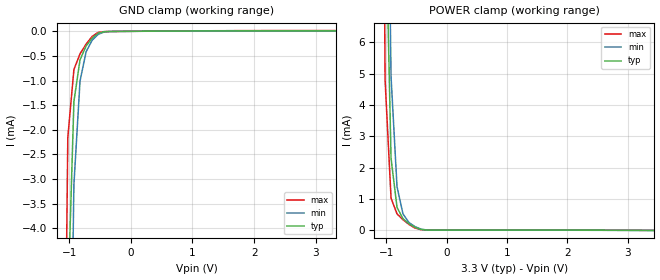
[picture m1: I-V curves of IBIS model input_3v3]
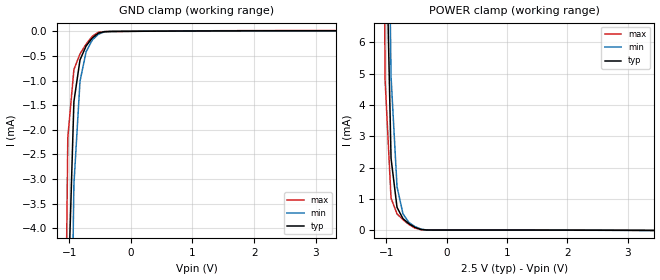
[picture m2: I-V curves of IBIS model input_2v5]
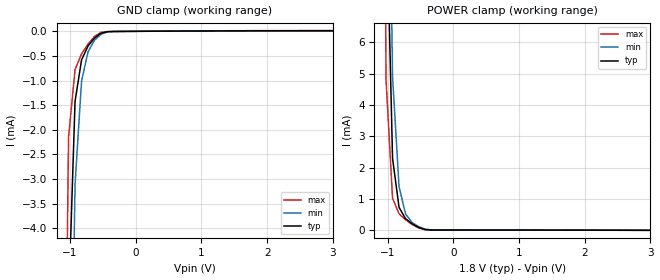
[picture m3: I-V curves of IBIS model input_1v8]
[IBIS ver]   4.1
[File name]   551s.ibs
|[File Rev]   1.0
|[Date]   March  3rd, 2016
[File Rev]   1.0
[Date]   April 25th, 2016[Source]   IDT
[Notes]   1. Temp typ=55C, min=80C, max=-40C
[Disclaimer]
READ THESE TERMS AND CONDITIONS CAREFULLY BEFORE USING THIS IBIS MODEL.  BY
USING THIS IBIS MODEL, YOU ARE ACCEPTING AND AGREEING TO THESE TERMS AND
CONDITIONS OF USE.
INTEGRATED DEVICE TECHNOLOGY, INC. ("IDT") HEREBY GRANTS THE USER OF THIS
IBIS MODEL ("USER") A NON-EXCLUSIVE, NONTRANSFERABLE LICENSE TO USE THIS
IBIS MODEL UNDER THE FOLLOWING TERMS: THE USER IS GRANTED THIS LICENSE ONLY
TO USE THE IBIS MODEL FOR DEMONSTRATION PURPOSES ONLY AND IS NOT GRANTED
RIGHTS TO SELL, COPY (EXCEPT AS NEEDED TO RUN THE IBIS MODEL), RENT, LEASE
OR SUB-LICENSE (EXCEPT FOR DEMONSTRATION) THE IBIS MODEL IN WHOLE OR IN
PART, OR IN MODIFIED FORM TO ANYONE. THE USER MAY MODIFY THE IBIS MODEL TO
SUIT ITS SPECIFIC APPLICATIONS, BUT  RIGHTS TO DERIVATIVE WORKS AND SUCH
MODIFICATIONS SHALL BELONG TO IDT.
THIS IBIS MODEL IS PROVIDED ON AN AS IS" BASIS AND IDT  MAKES ABSOLUTELY NO
WARRANTY WITH RESPECT TO THE INFORMATION CONTAINED HEREIN.  IDT DISCLAIMS
AND USER WAIVES ALL WARRANTIES, EXPRESS AND IMPLIED, INCLUDING WARRANTIES OF
MERCHANTABILITY AND FITNESS FOR A PARTICULAR PURPOSE.  THE ENTIRE RISK AS TO
QUALITY AND PERFORMANCE IS WITH THE USER  ACCORDINGLY, IN NO EVENT SHALL IDT
BE LIABLE FOR ANY DIRECT OR INDIRECT DAMAGES, WHETHER IN CONTRACT OR TORT,
INCLUDING ANY LOST PROFITS OR OTHER INCIDENTAL, CONSEQUENTIAL, EXEMPLARY, OR
PUNITIVE DAMAGES ARISING OUT OF THE USE OR APPLICATION OF THE  IBIS MODEL,
WHETHER OR NOT IDT HAD NOTICE OF SUCH DAMAGES.
IDT RESERVES THE RIGHT TO MAKE CHANGES WITHOUT NOTICE TO ANY PRODUCT HEREIN
TO IMPROVE RELIABILITY, FUNCTION, OR DESIGN. IDT DOES NOT CONVEY ANY LICENSE
UNDER PATENT RIGHTS OR ANY OTHER INTELLECTUAL PROPERTY RIGHTS, INCLUDING
THOSE OF THIRD PARTIES. IDT IS NOT OBLIGATED TO PROVIDE  MAINTENANCE OR
SUPPORT FOR THE LICENSED IBIS MODEL.
This model is for  IDT Fan Out Buffer
[Copyright]
Copyright 2002, Integrated Device Technology, Inc. All rights  reserved.
|History
|Rev 1.0 Created on April 25th, 2016
|   Component 551S
[Component]   551S
[Manufacturer]   Integrated Device Technology Inc.
[Package]
| Following package parameters are for the 8 pin DFN package (cmg_8)
| variable   typ   min   max
R_pkg   72.4655m   58.886m   86.045m
L_pkg   1.47175nH   1.11650nH   1.77850nH
C_pkg   0.07747pF   0.07444pF   0.08050pF
[Pin]  signal_name   model_name
1   ICLK   cmos_input
2   Q1   lvcmos
3   Q2   lvcmos
4   Q3   lvcmos
5   Q1   lvcmos
6   GND   gnd
7   VDD   POWER
8   OE   cmos_input
[Model Selector] lvcmos
lvcmos_3v3   3.3v cmos
lvcmos_2v5   2.5v cmos
lvcmos_1v8   1.8v cmos
[Model Selector] cmos_input
input_3v3  3.3v cmos
input_2v5  2.5v cmos
input_1v8  1.8v cmos
| Models and submodels in the file (6): input_3v3 (Input), input_2v5 (Input), input_1v8 (Input), lvcmos_3v3 (Output), lvcmos_2v5 (Output), lvcmos_1v8 (Output)
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|   Model INPUT_3V3
[Model]   input_3v3
Model_type   Input
Polarity   Non-Inverting
Vinl = 0.8V
Vinh = 2.0V
|   typ   min   max
C_comp   2pF   1.5pF   2.5pF
|   typ   min   max
[Voltage range]   3.3V   3.135V   3.465V
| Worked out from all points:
|   GND clamp passes 1 mA (typ) near -0.87 V on its own axis
|   POWER clamp passes 1 mA (typ) near -0.84 V on its own axis
[GND_clamp]
|Voltage   I (typ)   I (min)   I (max)
-3.3V     -5.877A    -5.408A    -6.492A
-1.122V   -26.71mA   -42.1mA    -13.37mA
-1.023V   -5.55mA    -11.5mA    -2.155mA
-924mV    -1.425mA   -3.112mA   -776.1uA
-825mV    -579.5uA   -1.011mA   -457.9uA
-726mV    -298.2uA   -414.7uA   -259.6uA
-627mV    -135.7uA   -178.7uA   -102.9uA
-528mV    -37.47uA   -59.22uA   -19.83uA
-429mV    -6.866uA   -11.92uA   -5.643uA
-330mV    -3.062uA   -3.056uA   -3.933uA
3.333V    11.06uA    8.259uA    15.61uA
| 3.43200e+00   1.10646e-05   9.85198e-06   1.56123e-05
| 3.46500e+00   1.10748e-05   1.56686e-05   1.56145e-05
| 3.53100e+00   1.10953e-05   2.73017e-05   1.56184e-05
| 3.63000e+00   1.22240e-05   9.00221e-05   1.56239e-05
| 3.72900e+00   2.94089e-05   2.01383e-04   1.56343e-05
| 3.82800e+00   9.82853e-05   4.04552e-04   1.61859e-05
| 3.92700e+00   2.13921e-04   9.74740e-04   3.14030e-05
| 4.02600e+00   3.75114e-04   3.15078e-03   1.08238e-04
| 4.12500e+00   7.35643e-04   1.23144e-02   2.36650e-04
| 4.22400e+00   2.30231e-03   4.64533e-02   3.97348e-04
| 4.32300e+00   1.10342e-02   1.34572e-01   6.21132e-04
| 4.42200e+00   5.26801e-02   2.82717e-01   1.53968e-03
| 4.52100e+00   1.68112e-01   4.72773e-01   9.44647e-03
| 4.62000e+00   3.53430e-01   6.87934e-01   6.47105e-02
| 4.71900e+00   5.79768e-01   9.19142e-01   2.25514e-01
| 4.81800e+00   8.28544e-01   1.16053e+00   4.62411e-01
| 4.91700e+00   1.09117e+00   1.40901e+00   7.35436e-01
| 5.01600e+00   1.36245e+00   1.66266e+00   1.02689e+00
| 5.11500e+00   1.63974e+00   1.92021e+00   1.32900e+00
| 5.21400e+00   1.92140e+00   2.18081e+00   1.63813e+00
| 5.31300e+00   2.20638e+00   2.44384e+00   1.95201e+00
| 5.41200e+00   2.49395e+00   2.70886e+00   2.26936e+00
| 5.51100e+00   2.78359e+00   2.97552e+00   2.58936e+00
| 5.61000e+00   3.07492e+00   3.24357e+00   2.91142e+00
| 5.70900e+00   3.36767e+00   3.51280e+00   3.23516e+00
| 5.80800e+00   3.66160e+00   3.78306e+00   3.56026e+00
| 5.90700e+00   3.95656e+00   4.05420e+00   3.88650e+00
| 6.00600e+00   4.25239e+00   4.32613e+00   4.21370e+00
| 6.10500e+00   4.54899e+00   4.59875e+00   4.54174e+00
| 6.20400e+00   4.84627e+00   4.87198e+00   4.87049e+00
| 6.30300e+00   5.14414e+00   5.14577e+00   5.19987e+00
| 6.40200e+00   5.44256e+00   5.42005e+00   5.52980e+00
| 6.50100e+00   5.74145e+00   5.69479e+00   5.86022e+00
| 6.60000e+00   6.04077e+00   5.96994e+00   6.19109e+00
[Power_clamp]
|Voltage   I (typ)   I (min)   I (max)
-3.3V     6.041A     5.512A     6.743A
-1.122V   52.68mA    68.73mA    36.05mA
-1.023V   11.03mA    19.49mA    4.811mA
-924mV    2.302mA    4.908mA    1.028mA
-825mV    735.6uA    1.396mA    528.4uA
-726mV    375.1uA    526.2uA    340.6uA
-627mV    213.9uA    252.9uA    189.6uA
-528mV    98.2uA     121.6uA    75.41uA
-429mV    29.41uA    42.52uA    21.55uA
-231mV    11.1uA     8.404uA    15.63uA
3.432V    -1.145uA   -2.375uA   378.6nA
|   Model INPUT_2V5
[Model]   input_2v5
Model_type Input
Vinl =   0.9500V
Vinh =   1.5500V
C_comp   2.0000pF   1.5000pF   2.5000pF
[Temperature Range]   55.0000   80.0000   -40.0000
[Voltage Range]   2.5000V   2.3750V   2.6250V
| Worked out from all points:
|   GND clamp passes 1 mA (typ) near -0.87 V on its own axis
|   POWER clamp passes 1 mA (typ) near -0.84 V on its own axis
[GND_clamp]
|Voltage   I (typ)   I (min)   I (max)
-3.3V     -5.877A    -5.408A    -6.492A
-1.122V   -26.71mA   -42.1mA    -13.37mA
-1.023V   -5.55mA    -11.5mA    -2.155mA
-924mV    -1.425mA   -3.112mA   -776.1uA
-825mV    -579.5uA   -1.011mA   -457.9uA
-726mV    -298.2uA   -414.7uA   -259.6uA
-627mV    -135.7uA   -178.7uA   -102.9uA
-528mV    -37.47uA   -59.22uA   -19.83uA
-429mV    -6.866uA   -11.92uA   -5.643uA
-330mV    -3.062uA   -3.056uA   -3.933uA
3.333V    11.06uA    8.259uA    15.61uA
| 3.43200e+00   1.10646e-05   9.85198e-06   1.56123e-05
| 3.46500e+00   1.10748e-05   1.56686e-05   1.56145e-05
| 3.53100e+00   1.10953e-05   2.73017e-05   1.56184e-05
| 3.63000e+00   1.22240e-05   9.00221e-05   1.56239e-05
| 3.72900e+00   2.94089e-05   2.01383e-04   1.56343e-05
| 3.82800e+00   9.82853e-05   4.04552e-04   1.61859e-05
| 3.92700e+00   2.13921e-04   9.74740e-04   3.14030e-05
| 4.02600e+00   3.75114e-04   3.15078e-03   1.08238e-04
| 4.12500e+00   7.35643e-04   1.23144e-02   2.36650e-04
| 4.22400e+00   2.30231e-03   4.64533e-02   3.97348e-04
| 4.32300e+00   1.10342e-02   1.34572e-01   6.21132e-04
| 4.42200e+00   5.26801e-02   2.82717e-01   1.53968e-03
| 4.52100e+00   1.68112e-01   4.72773e-01   9.44647e-03
| 4.62000e+00   3.53430e-01   6.87934e-01   6.47105e-02
| 4.71900e+00   5.79768e-01   9.19142e-01   2.25514e-01
| 4.81800e+00   8.28544e-01   1.16053e+00   4.62411e-01
| 4.91700e+00   1.09117e+00   1.40901e+00   7.35436e-01
| 5.01600e+00   1.36245e+00   1.66266e+00   1.02689e+00
| 5.11500e+00   1.63974e+00   1.92021e+00   1.32900e+00
| 5.21400e+00   1.92140e+00   2.18081e+00   1.63813e+00
| 5.31300e+00   2.20638e+00   2.44384e+00   1.95201e+00
| 5.41200e+00   2.49395e+00   2.70886e+00   2.26936e+00
| 5.51100e+00   2.78359e+00   2.97552e+00   2.58936e+00
| 5.61000e+00   3.07492e+00   3.24357e+00   2.91142e+00
| 5.70900e+00   3.36767e+00   3.51280e+00   3.23516e+00
| 5.80800e+00   3.66160e+00   3.78306e+00   3.56026e+00
| 5.90700e+00   3.95656e+00   4.05420e+00   3.88650e+00
| 6.00600e+00   4.25239e+00   4.32613e+00   4.21370e+00
| 6.10500e+00   4.54899e+00   4.59875e+00   4.54174e+00
| 6.20400e+00   4.84627e+00   4.87198e+00   4.87049e+00
| 6.30300e+00   5.14414e+00   5.14577e+00   5.19987e+00
| 6.40200e+00   5.44256e+00   5.42005e+00   5.52980e+00
| 6.50100e+00   5.74145e+00   5.69479e+00   5.86022e+00
| 6.60000e+00   6.04077e+00   5.96994e+00   6.19109e+00
[Power_clamp]
|Voltage   I (typ)   I (min)   I (max)
-3.3V     6.041A     5.512A     6.743A
-1.122V   52.68mA    68.73mA    36.05mA
-1.023V   11.03mA    19.49mA    4.811mA
-924mV    2.302mA    4.908mA    1.028mA
-825mV    735.6uA    1.396mA    528.4uA
-726mV    375.1uA    526.2uA    340.6uA
-627mV    213.9uA    252.9uA    189.6uA
-528mV    98.2uA     121.6uA    75.41uA
-429mV    29.41uA    42.52uA    21.55uA
-231mV    11.1uA     8.404uA    15.63uA
3.432V    -1.145uA   -2.375uA   378.6nA
|   Model INPUT_1V8
[Model]   input_1v8
Model_type Input
Vinl =   0.6000V
Vinh =   1.2000V
C_comp   2.0000pF   1.5000pF   2.5000pF
[Temperature Range]   55.0000   80.0000   -40.0000
[Voltage Range]   1.8000V   1.7100V   1.8900V
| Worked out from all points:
|   GND clamp passes 1 mA (typ) near -0.87 V on its own axis
|   POWER clamp passes 1 mA (typ) near -0.84 V on its own axis
[GND_clamp]
|Voltage   I (typ)   I (min)   I (max)
-3.3V     -5.877A    -5.408A    -6.492A
-1.122V   -26.71mA   -42.1mA    -13.37mA
-1.023V   -5.55mA    -11.5mA    -2.155mA
-924mV    -1.425mA   -3.112mA   -776.1uA
-825mV    -579.5uA   -1.011mA   -457.9uA
-726mV    -298.2uA   -414.7uA   -259.6uA
-627mV    -135.7uA   -178.7uA   -102.9uA
-528mV    -37.47uA   -59.22uA   -19.83uA
-429mV    -6.866uA   -11.92uA   -5.643uA
-330mV    -3.062uA   -3.056uA   -3.933uA
3.333V    11.06uA    8.259uA    15.61uA
| 3.43200e+00   1.10646e-05   9.85198e-06   1.56123e-05
| 3.46500e+00   1.10748e-05   1.56686e-05   1.56145e-05
| 3.53100e+00   1.10953e-05   2.73017e-05   1.56184e-05
| 3.63000e+00   1.22240e-05   9.00221e-05   1.56239e-05
| 3.72900e+00   2.94089e-05   2.01383e-04   1.56343e-05
| 3.82800e+00   9.82853e-05   4.04552e-04   1.61859e-05
| 3.92700e+00   2.13921e-04   9.74740e-04   3.14030e-05
| 4.02600e+00   3.75114e-04   3.15078e-03   1.08238e-04
| 4.12500e+00   7.35643e-04   1.23144e-02   2.36650e-04
| 4.22400e+00   2.30231e-03   4.64533e-02   3.97348e-04
| 4.32300e+00   1.10342e-02   1.34572e-01   6.21132e-04
| 4.42200e+00   5.26801e-02   2.82717e-01   1.53968e-03
| 4.52100e+00   1.68112e-01   4.72773e-01   9.44647e-03
| 4.62000e+00   3.53430e-01   6.87934e-01   6.47105e-02
| 4.71900e+00   5.79768e-01   9.19142e-01   2.25514e-01
| 4.81800e+00   8.28544e-01   1.16053e+00   4.62411e-01
| 4.91700e+00   1.09117e+00   1.40901e+00   7.35436e-01
| 5.01600e+00   1.36245e+00   1.66266e+00   1.02689e+00
| 5.11500e+00   1.63974e+00   1.92021e+00   1.32900e+00
| 5.21400e+00   1.92140e+00   2.18081e+00   1.63813e+00
| 5.31300e+00   2.20638e+00   2.44384e+00   1.95201e+00
| 5.41200e+00   2.49395e+00   2.70886e+00   2.26936e+00
| 5.51100e+00   2.78359e+00   2.97552e+00   2.58936e+00
| 5.61000e+00   3.07492e+00   3.24357e+00   2.91142e+00
| 5.70900e+00   3.36767e+00   3.51280e+00   3.23516e+00
| 5.80800e+00   3.66160e+00   3.78306e+00   3.56026e+00
| 5.90700e+00   3.95656e+00   4.05420e+00   3.88650e+00
| 6.00600e+00   4.25239e+00   4.32613e+00   4.21370e+00
| 6.10500e+00   4.54899e+00   4.59875e+00   4.54174e+00
| 6.20400e+00   4.84627e+00   4.87198e+00   4.87049e+00
| 6.30300e+00   5.14414e+00   5.14577e+00   5.19987e+00
| 6.40200e+00   5.44256e+00   5.42005e+00   5.52980e+00
| 6.50100e+00   5.74145e+00   5.69479e+00   5.86022e+00
| 6.60000e+00   6.04077e+00   5.96994e+00   6.19109e+00
[Power_clamp]
|Voltage   I (typ)   I (min)   I (max)
-3.3V     6.041A     5.512A     6.743A
-1.122V   52.68mA    68.73mA    36.05mA
-1.023V   11.03mA    19.49mA    4.811mA
-924mV    2.302mA    4.908mA    1.028mA
-825mV    735.6uA    1.396mA    528.4uA
-726mV    375.1uA    526.2uA    340.6uA
-627mV    213.9uA    252.9uA    189.6uA
-528mV    98.2uA     121.6uA    75.41uA
-429mV    29.41uA    42.52uA    21.55uA
-231mV    11.1uA     8.404uA    15.63uA
3.432V    -1.145uA   -2.375uA   378.6nA
